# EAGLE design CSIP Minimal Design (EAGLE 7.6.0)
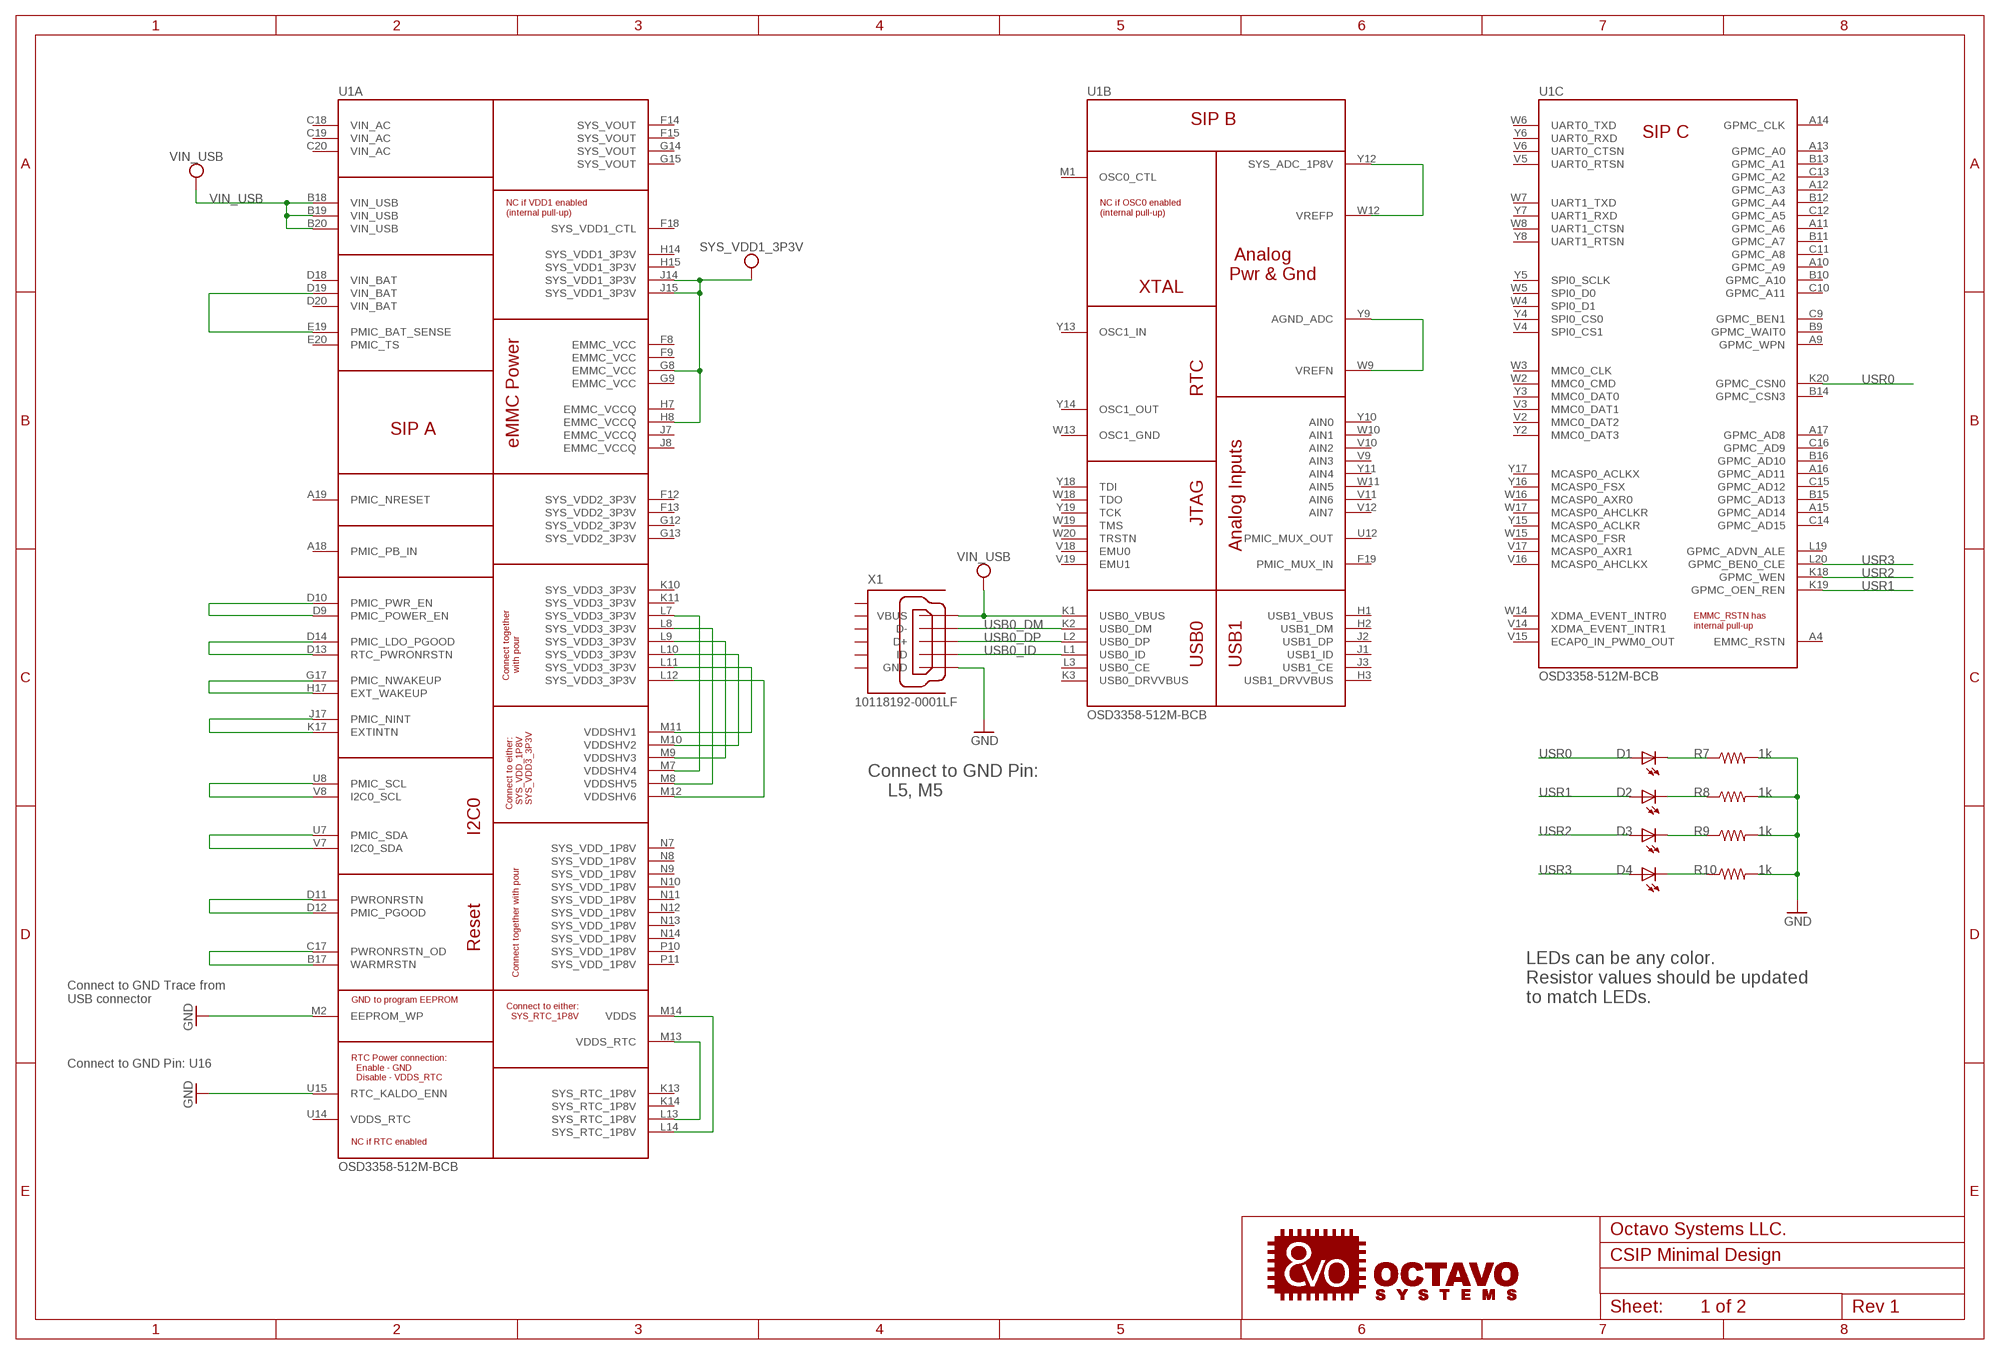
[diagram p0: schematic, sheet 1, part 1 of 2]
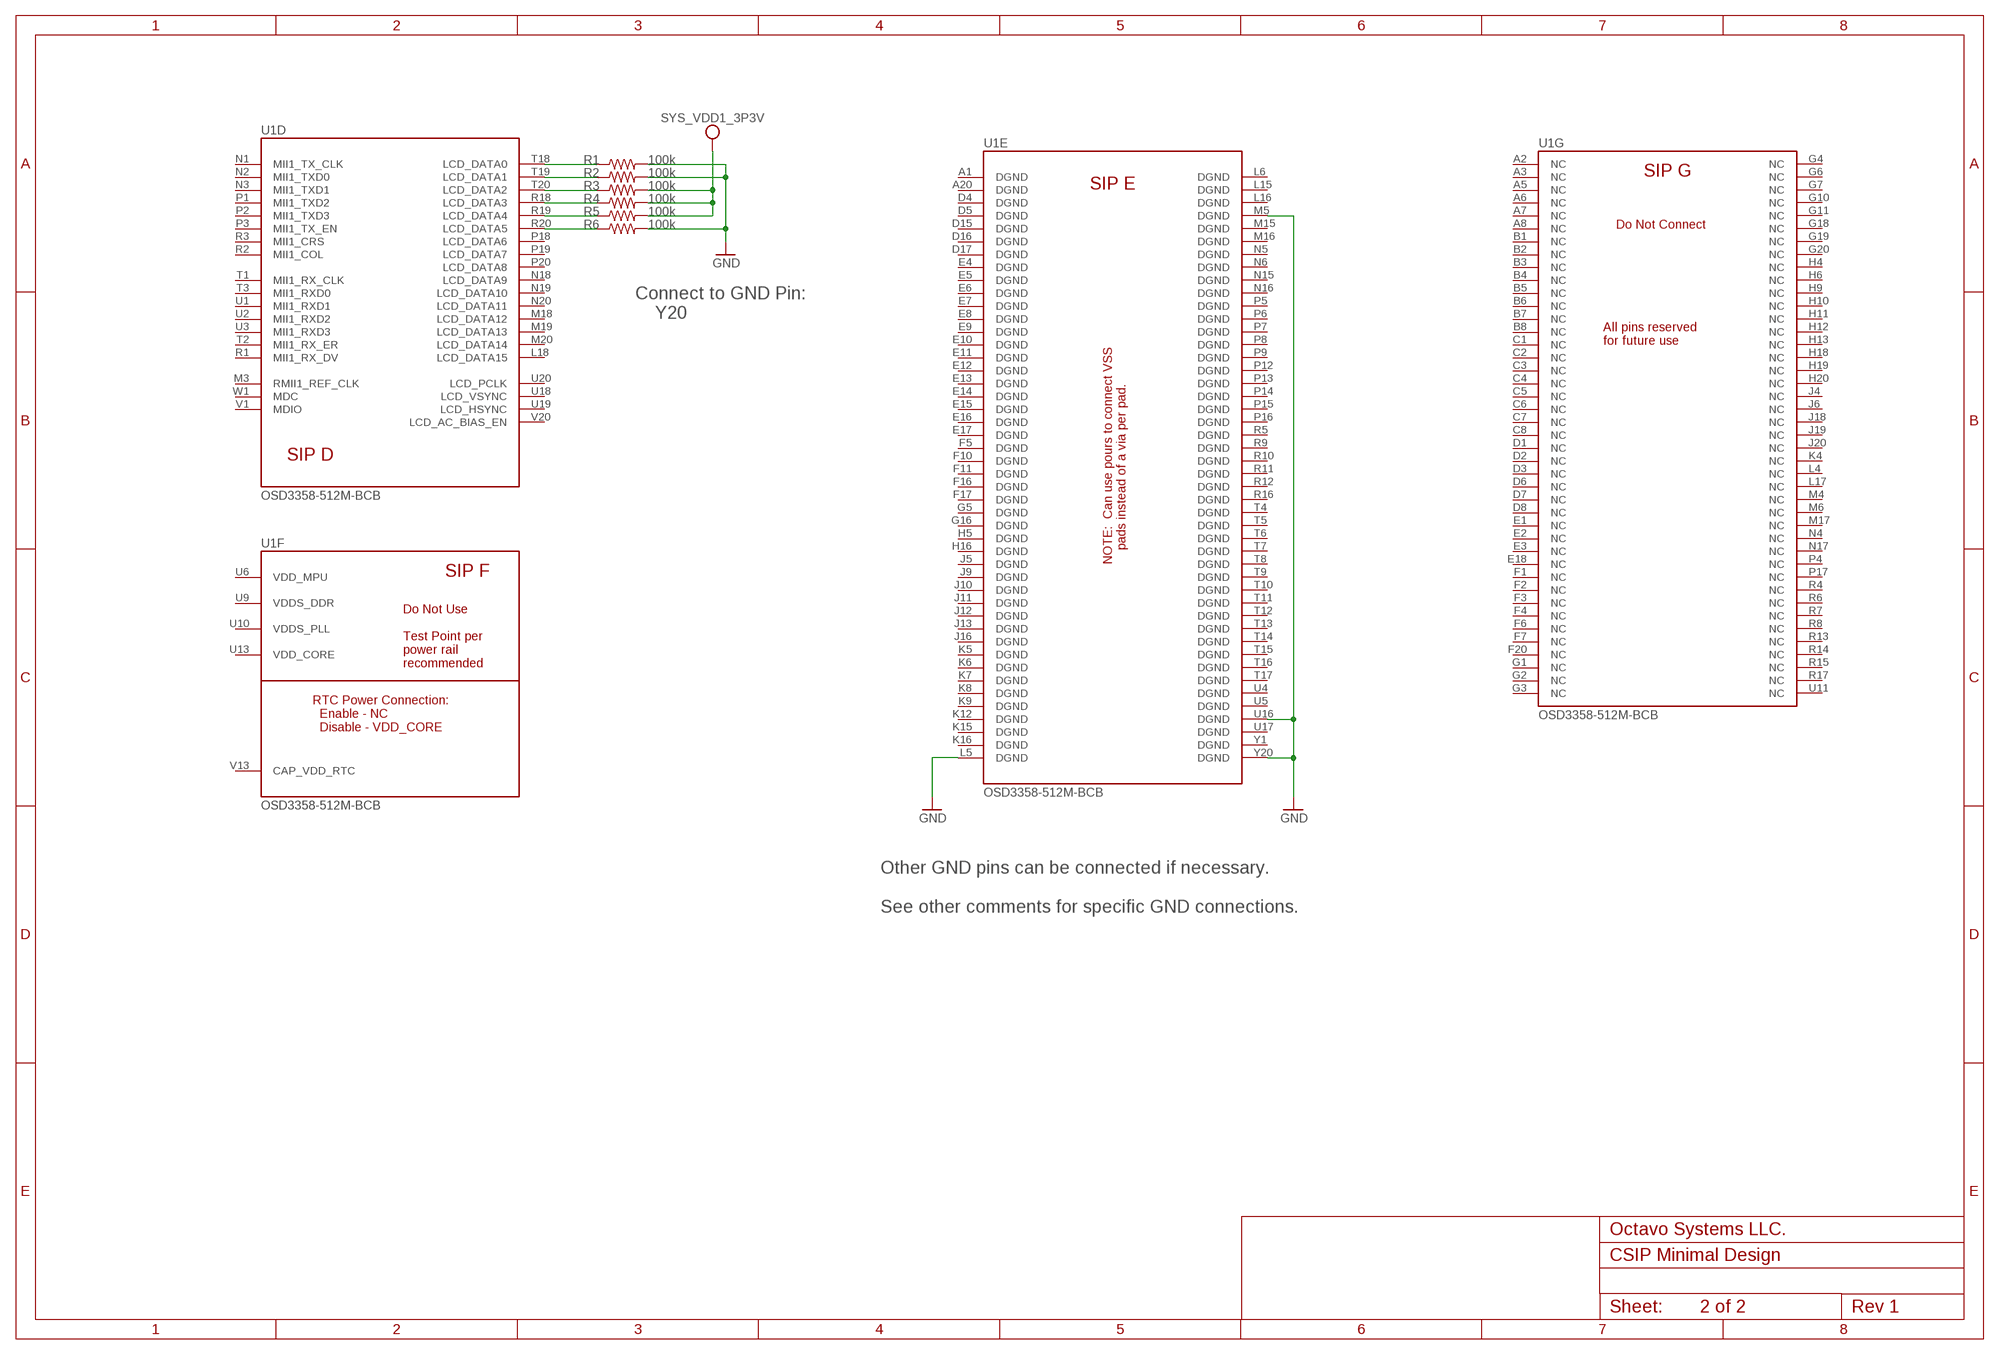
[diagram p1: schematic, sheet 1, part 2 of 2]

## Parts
D1  LTST-C191TBKTLED_EIA-STD  [EIA-STD]
D2  LTST-C191TBKTLED_EIA-STD  [EIA-STD]
D3  LTST-C191TBKTLED_EIA-STD  [EIA-STD]
D4  LTST-C191TBKTLED_EIA-STD  [EIA-STD]
R1  100k  R-US_R0402  [R0402]
R2  100k  R-US_R0402  [R0402]
R3  100k  R-US_R0402  [R0402]
R4  100k  R-US_R0402  [R0402]
R5  100k  R-US_R0402  [R0402]
R6  100k  R-US_R0402  [R0402]
R7  1k  R-US_R0402  [R0402]
R8  1k  R-US_R0402  [R0402]
R9  1k  R-US_R0402  [R0402]
R10  1k  R-US_R0402  [R0402]
U1  OSD3358-512M-BCB  [OSD335X-BGA-400]
X1  10118192-0001LF  [10118192-0001LF(MICRO-USB-B-AMPHENOL-FCI)]

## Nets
GND: R1.2 R2.2 R6.2 R7.2 R8.2 R9.2 R10.2 U1.L5(E:DGND) U1.M2(A:EEPROM_WP) U1.M5(E:DGND) U1.U15(A:RTC_KALDO_ENN) U1.U16(E:DGND) U1.Y20(E:DGND) X1.GND
N$1: U1.G17(A:PMIC_NWAKEUP) U1.H17(A:EXT_WAKEUP)
N$2: U1.D13(A:RTC_PWRONRSTN) U1.D14(A:PMIC_LDO_PGOOD)
N$3: U1.D9(A:PMIC_POWER_EN) U1.D10(A:PMIC_PWR_EN)
N$4: U1.J17(A:PMIC_NINT) U1.K17(A:EXTINTN)
N$5: U1.U8(A:PMIC_SCL) U1.V8(A:I2C0_SCL)
N$6: U1.U7(A:PMIC_SDA) U1.V7(A:I2C0_SDA)
N$7: U1.L13(A:SYS_RTC_1P8V) U1.M13(A:VDDS_RTC)
N$9: U1.D11(A:PWRONRSTN) U1.D12(A:PMIC_PGOOD)
N$10: U1.B17(A:WARMRSTN) U1.C17(A:PWRONRSTN_OD)
N$11: U1.W12(B:VREFP) U1.Y12(B:SYS_ADC_1P8V)
N$13: U1.W9(B:VREFN) U1.Y9(B:AGND_ADC)
N$14: R1.1 U1.T18(D:LCD_DATA0)
N$15: R2.1 U1.T19(D:LCD_DATA1)
N$16: U1.L11(A:SYS_VDD3_3P3V) U1.M11(A:VDDSHV1)
N$17: U1.L10(A:SYS_VDD3_3P3V) U1.M10(A:VDDSHV2)
N$18: R3.1 U1.T20(D:LCD_DATA2)
N$19: R4.1 U1.R18(D:LCD_DATA3)
N$20: R5.1 U1.R19(D:LCD_DATA4)
N$21: R6.1 U1.R20(D:LCD_DATA5)
N$22: U1.L9(A:SYS_VDD3_3P3V) U1.M9(A:VDDSHV3)
N$23: U1.L7(A:SYS_VDD3_3P3V) U1.M7(A:VDDSHV4)
N$24: U1.L8(A:SYS_VDD3_3P3V) U1.M8(A:VDDSHV5)
N$25: D1.2(C) R7.1
N$26: D2.2(C) R8.1
N$27: D3.2(C) R9.1
N$28: D4.2(C) R10.1
SYS_RTC_1P8V: U1.L14(A:SYS_RTC_1P8V) U1.M14(A:VDDS)
SYS_VDD1_3P3V: R3.2 R4.2 R5.2 U1.G8(A:EMMC_VCC) U1.H8(A:EMMC_VCCQ) U1.J14(A:SYS_VDD1_3P3V) U1.J15(A:SYS_VDD1_3P3V)
SYS_VDD3_3P3V: U1.L12(A:SYS_VDD3_3P3V) U1.M12(A:VDDSHV6)
USB0_DM: U1.K2(B:USB0_DM) X1.D-
USB0_DP: U1.L2(B:USB0_DP) X1.D+
USB0_ID: U1.L1(B:USB0_ID) X1.ID
USR0: D1.1(A) U1.K20(C:GPMC_CSN0)
USR1: D2.1(A) U1.K19(C:GPMC_OEN_REN)
USR2: D3.1(A) U1.K18(C:GPMC_WEN)
USR3: D4.1(A) U1.L20(C:GPMC_BEN0_CLE)
VIN_BAT: U1.D19(A:VIN_BAT) U1.E19(A:PMIC_BAT_SENSE)
VIN_USB: U1.B18(A:VIN_USB) U1.B19(A:VIN_USB) U1.B20(A:VIN_USB) U1.K1(B:USB0_VBUS) X1.VBUS
Unconnected: U1.A1(E:DGND) U1.A2(G:NC) U1.A3(G:NC) U1.A4(C:EMMC_RSTN) U1.A5(G:NC) U1.A6(G:NC) U1.A7(G:NC) U1.A8(G:NC) U1.A9(C:GPMC_WPN) U1.A10(C:GPMC_A9) U1.A11(C:GPMC_A6) U1.A12(C:GPMC_A3) U1.A13(C:GPMC_A0) U1.A14(C:GPMC_CLK) U1.A15(C:GPMC_AD14) U1.A16(C:GPMC_AD11) U1.A17(C:GPMC_AD8) U1.A18(A:PMIC_PB_IN) U1.A19(A:PMIC_NRESET) U1.A20(E:DGND) U1.B1(G:NC) U1.B2(G:NC) U1.B3(G:NC) U1.B4(G:NC) U1.B5(G:NC) U1.B6(G:NC) U1.B7(G:NC) U1.B8(G:NC) U1.B9(C:GPMC_WAIT0) U1.B10(C:GPMC_A10) U1.B11(C:GPMC_A7) U1.B12(C:GPMC_A4) U1.B13(C:GPMC_A1) U1.B14(C:GPMC_CSN3) U1.B15(C:GPMC_AD13) U1.B16(C:GPMC_AD10) U1.C1(G:NC) U1.C2(G:NC) U1.C3(G:NC) U1.C4(G:NC) U1.C5(G:NC) U1.C6(G:NC) U1.C7(G:NC) U1.C8(G:NC) U1.C9(C:GPMC_BEN1) U1.C10(C:GPMC_A11) U1.C11(C:GPMC_A8) U1.C12(C:GPMC_A5) U1.C13(C:GPMC_A2) U1.C14(C:GPMC_AD15) U1.C15(C:GPMC_AD12) U1.C16(C:GPMC_AD9) U1.D1(G:NC) U1.D2(G:NC) U1.D3(G:NC) U1.D4(E:DGND) U1.D5(E:DGND) U1.D6(G:NC) U1.D7(G:NC) U1.D8(G:NC) U1.D15(E:DGND) U1.D16(E:DGND) U1.D17(E:DGND) U1.E1(G:NC) U1.E2(G:NC) U1.E3(G:NC) U1.E4(E:DGND) U1.E5(E:DGND) U1.E6(E:DGND) U1.E7(E:DGND) U1.E8(E:DGND) U1.E9(E:DGND) U1.E10(E:DGND) U1.E11(E:DGND) U1.E12(E:DGND) U1.E13(E:DGND) U1.E14(E:DGND) U1.E15(E:DGND) U1.E16(E:DGND) U1.E17(E:DGND) U1.E18(G:NC) U1.E20(A:PMIC_TS) U1.F1(G:NC) U1.F2(G:NC) U1.F3(G:NC) U1.F4(G:NC) U1.F5(E:DGND) U1.F6(G:NC) U1.F7(G:NC) U1.F8(A:EMMC_VCC) U1.F9(A:EMMC_VCC) U1.F10(E:DGND) U1.F11(E:DGND) U1.F16(E:DGND) U1.F17(E:DGND) U1.F18(A:SYS_VDD1_CTL) U1.F19(B:PMIC_MUX_IN) U1.F20(G:NC) U1.G1(G:NC) U1.G2(G:NC) U1.G3(G:NC) U1.G4(G:NC) U1.G5(E:DGND) U1.G6(G:NC) U1.G7(G:NC) U1.G9(A:EMMC_VCC) U1.G10(G:NC) U1.G11(G:NC) U1.G16(E:DGND) U1.G18(G:NC) U1.G19(G:NC) U1.G20(G:NC) U1.H1(B:USB1_VBUS) U1.H2(B:USB1_DM) U1.H3(B:USB1_DRVVBUS) U1.H4(G:NC) U1.H5(E:DGND) U1.H6(G:NC) U1.H7(A:EMMC_VCCQ) U1.H9(G:NC) U1.H10(G:NC) U1.H11(G:NC) U1.H12(G:NC) U1.H13(G:NC) U1.H16(E:DGND) U1.H18(G:NC) U1.H19(G:NC) U1.H20(G:NC) U1.J1(B:USB1_ID) U1.J2(B:USB1_DP) U1.J3(B:USB1_CE) U1.J4(G:NC) U1.J5(E:DGND) U1.J6(G:NC) U1.J7(A:EMMC_VCCQ) U1.J8(A:EMMC_VCCQ) U1.J9(E:DGND) U1.J10(E:DGND) U1.J11(E:DGND) U1.J12(E:DGND) U1.J13(E:DGND) U1.J16(E:DGND) U1.J18(G:NC) U1.J19(G:NC) U1.J20(G:NC) U1.K3(B:USB0_DRVVBUS) U1.K4(G:NC) U1.K5(E:DGND) U1.K6(E:DGND) U1.K7(E:DGND) U1.K8(E:DGND) U1.K9(E:DGND) U1.K12(E:DGND) U1.K15(E:DGND) U1.K16(E:DGND) U1.L3(B:USB0_CE) U1.L4(G:NC) U1.L6(E:DGND) U1.L15(E:DGND) U1.L16(E:DGND) U1.L17(G:NC) U1.L18(D:LCD_DATA15) U1.L19(C:GPMC_ADVN_ALE) U1.M1(B:OSC0_CTL) U1.M3(D:RMII1_REF_CLK) U1.M4(G:NC) U1.M6(G:NC) U1.M15(E:DGND) U1.M16(E:DGND) U1.M17(G:NC) U1.M18(D:LCD_DATA12) U1.M19(D:LCD_DATA13) U1.M20(D:LCD_DATA14) U1.N1(D:MII1_TX_CLK) U1.N2(D:MII1_TXD0) U1.N3(D:MII1_TXD1) U1.N4(G:NC) U1.N5(E:DGND) U1.N6(E:DGND) U1.N15(E:DGND) U1.N16(E:DGND) U1.N17(G:NC) U1.N18(D:LCD_DATA9) U1.N19(D:LCD_DATA10) U1.N20(D:LCD_DATA11) U1.P1(D:MII1_TXD2) U1.P2(D:MII1_TXD3) U1.P3(D:MII1_TX_EN) U1.P4(G:NC) U1.P5(E:DGND) U1.P6(E:DGND) U1.P7(E:DGND) U1.P8(E:DGND) U1.P9(E:DGND) U1.P12(E:DGND) U1.P13(E:DGND) U1.P14(E:DGND) U1.P15(E:DGND) U1.P16(E:DGND) U1.P17(G:NC) U1.P18(D:LCD_DATA6) U1.P19(D:LCD_DATA7) U1.P20(D:LCD_DATA8) U1.R1(D:MII1_RX_DV) U1.R2(D:MII1_COL) U1.R3(D:MII1_CRS) U1.R4(G:NC) U1.R5(E:DGND) U1.R6(G:NC) U1.R7(G:NC) U1.R8(G:NC) U1.R9(E:DGND) U1.R10(E:DGND) U1.R11(E:DGND) U1.R12(E:DGND) U1.R13(G:NC) U1.R14(G:NC) U1.R15(G:NC) U1.R16(E:DGND) U1.R17(G:NC) U1.T1(D:MII1_RX_CLK) U1.T2(D:MII1_RX_ER) U1.T3(D:MII1_RXD0) U1.T4(E:DGND) U1.T5(E:DGND) U1.T6(E:DGND) U1.T7(E:DGND) U1.T8(E:DGND) U1.T9(E:DGND) U1.T10(E:DGND) U1.T11(E:DGND) U1.T12(E:DGND) U1.T13(E:DGND) U1.T14(E:DGND) U1.T15(E:DGND) U1.T16(E:DGND) U1.T17(E:DGND) U1.U1(D:MII1_RXD1) U1.U2(D:MII1_RXD2) U1.U3(D:MII1_RXD3) U1.U4(E:DGND) U1.U5(E:DGND) U1.U6(F:VDD_MPU) U1.U9(F:VDDS_DDR) U1.U10(F:VDDS_PLL) U1.U11(G:NC) U1.U12(B:PMIC_MUX_OUT) U1.U13(F:VDD_CORE) U1.U14(A:VDDS_RTC) U1.U17(E:DGND) U1.U18(D:LCD_VSYNC) U1.U19(D:LCD_HSYNC) U1.U20(D:LCD_PCLK) U1.V1(D:MDIO) U1.V2(C:MMC0_DAT2) U1.V3(C:MMC0_DAT1) U1.V4(C:SPI0_CS1) U1.V5(C:UART0_RTSN) U1.V6(C:UART0_CTSN) U1.V9(B:AIN3) U1.V10(B:AIN2) U1.V11(B:AIN6) U1.V12(B:AIN7) U1.V13(F:CAP_VDD_RTC) U1.V14(C:XDMA_EVENT_INTR1) U1.V15(C:ECAP0_IN_PWM0_OUT) U1.V16(C:MCASP0_AHCLKX) U1.V17(C:MCASP0_AXR1) U1.V18(B:EMU0) U1.V19(B:EMU1) U1.V20(D:LCD_AC_BIAS_EN) U1.W1(D:MDC) U1.W2(C:MMC0_CMD) U1.W3(C:MMC0_CLK) U1.W4(C:SPI0_D1) U1.W5(C:SPI0_D0) U1.W6(C:UART0_TXD) U1.W7(C:UART1_TXD) U1.W8(C:UART1_CTSN) U1.W10(B:AIN1) U1.W11(B:AIN5) U1.W13(B:OSC1_GND) U1.W14(C:XDMA_EVENT_INTR0) U1.W15(C:MCASP0_FSR) U1.W16(C:MCASP0_AXR0) U1.W17(C:MCASP0_AHCLKR) U1.W18(B:TDO) U1.W19(B:TMS) U1.W20(B:TRSTN) U1.Y1(E:DGND) U1.Y2(C:MMC0_DAT3) U1.Y3(C:MMC0_DAT0) U1.Y4(C:SPI0_CS0) U1.Y5(C:SPI0_SCLK) U1.Y6(C:UART0_RXD) U1.Y7(C:UART1_RXD) U1.Y8(C:UART1_RTSN) U1.Y10(B:AIN0) U1.Y11(B:AIN4) U1.Y13(B:OSC1_IN) U1.Y14(B:OSC1_OUT) U1.Y15(C:MCASP0_ACLKR) U1.Y16(C:MCASP0_FSX) U1.Y17(C:MCASP0_ACLKX) U1.Y18(B:TDI) U1.Y19(B:TCK) X1.CGND1(SGND1) X1.CGND2(SGND2) X1.CGND3(SGND3) X1.CGND4(SGND4) X1.CGND5(SGND5) X1.CGND6(SGND6)

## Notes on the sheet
- Connect to GND Pin: 
      Y20
- Connect to GND Pin: 
      L5, M5
- Other GND pins can be connected if necessary.
  
  See other comments for specific GND connections.
- Connect to GND Trace from 
  USB connector
- LEDs can be any color.
  Resistor values should be updated 
  to match LEDs.
- Connect to GND Pin: U16
- 1 of 2 | 2 of 2

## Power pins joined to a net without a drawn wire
SYS_RTC_1P8V: U1.K13(A:SYS_RTC_1P8V) U1.K14(A:SYS_RTC_1P8V)
SYS_VDD1_3P3V: U1.H14(A:SYS_VDD1_3P3V) U1.H15(A:SYS_VDD1_3P3V)
SYS_VDD2_3P3V: U1.F12(A:SYS_VDD2_3P3V) U1.F13(A:SYS_VDD2_3P3V) U1.G12(A:SYS_VDD2_3P3V) U1.G13(A:SYS_VDD2_3P3V)
SYS_VDD3_3P3V: U1.K10(A:SYS_VDD3_3P3V) U1.K11(A:SYS_VDD3_3P3V)
SYS_VDD_1P8V: U1.N7(A:SYS_VDD_1P8V) U1.N8(A:SYS_VDD_1P8V) U1.N9(A:SYS_VDD_1P8V) U1.N10(A:SYS_VDD_1P8V) U1.N11(A:SYS_VDD_1P8V) U1.N12(A:SYS_VDD_1P8V) U1.N13(A:SYS_VDD_1P8V) U1.N14(A:SYS_VDD_1P8V) U1.P10(A:SYS_VDD_1P8V) U1.P11(A:SYS_VDD_1P8V)
SYS_VOUT: U1.F14(A:SYS_VOUT) U1.F15(A:SYS_VOUT) U1.G14(A:SYS_VOUT) U1.G15(A:SYS_VOUT)
VIN_AC: U1.C18(A:VIN_AC) U1.C19(A:VIN_AC) U1.C20(A:VIN_AC)
VIN_BAT: U1.D18(A:VIN_BAT) U1.D20(A:VIN_BAT)

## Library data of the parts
D1-D4 = OSD3358-SM-RED Platform:LTST-C191TBKT: PointLED® Enhanced Thinfilm LED TOP & BOTTOM mount
R1-R10 = OSD3358-SM IOT SoM:R-US_: RESISTOR, American symbol
U1 = Octavo-Systems:OSD3358-512M-BCB: Octavo Systems LLC OSD335x Family SiP: 27mm x 27mm, 1.27mm pitch 400 pin BGA contains AM3358, 512MB DDR3, TPS65217, TL5209, 4KB EEPROM, 4GB eMMC, 24MHz oscillator, and passives. Commerical Temperature (case): 0C to 85C.
X1 = OSD3358-SM-RED Platform:10118192-0001LF: Amphenol FCI Micro USB Type B Complete Surface Mount (SMT) no guide holes

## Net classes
1 ground: width 0.152 mm, drill 0.254 mm, clearance 0.152 mm
3 power: width 0.152 mm, drill 0.254 mm, clearance 0.152 mm

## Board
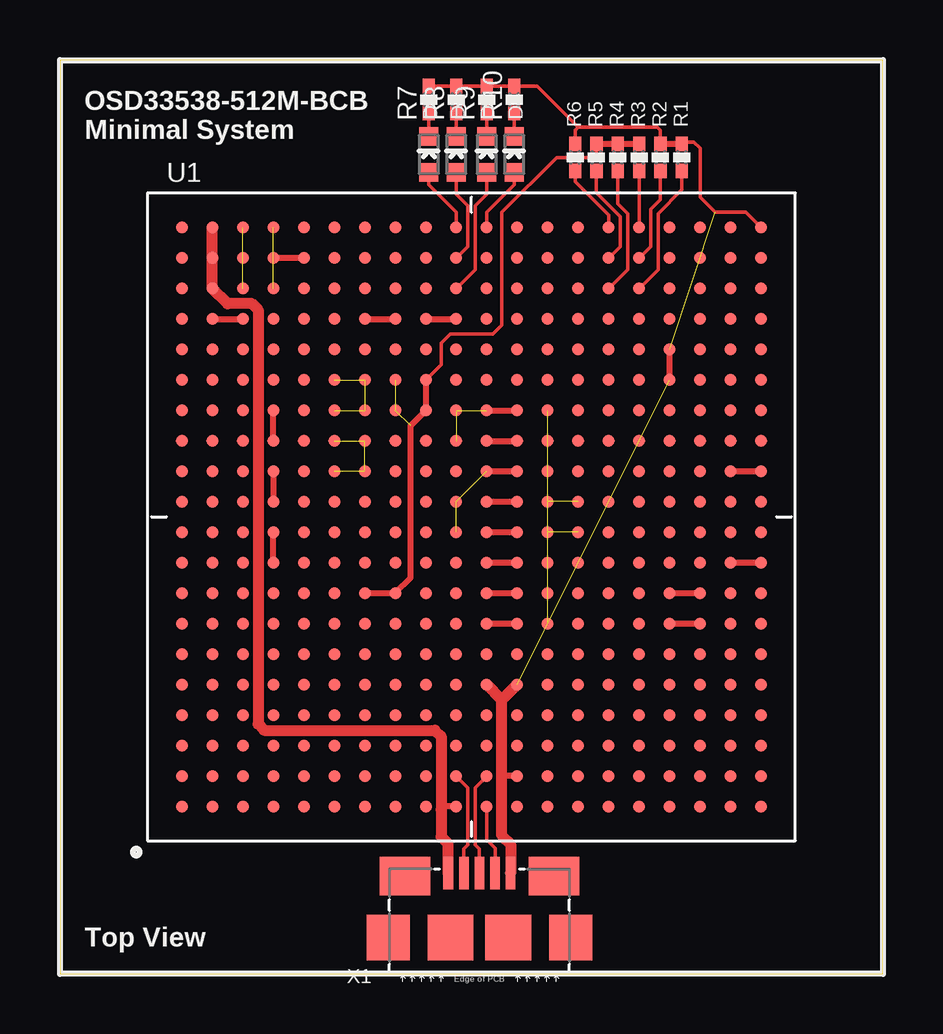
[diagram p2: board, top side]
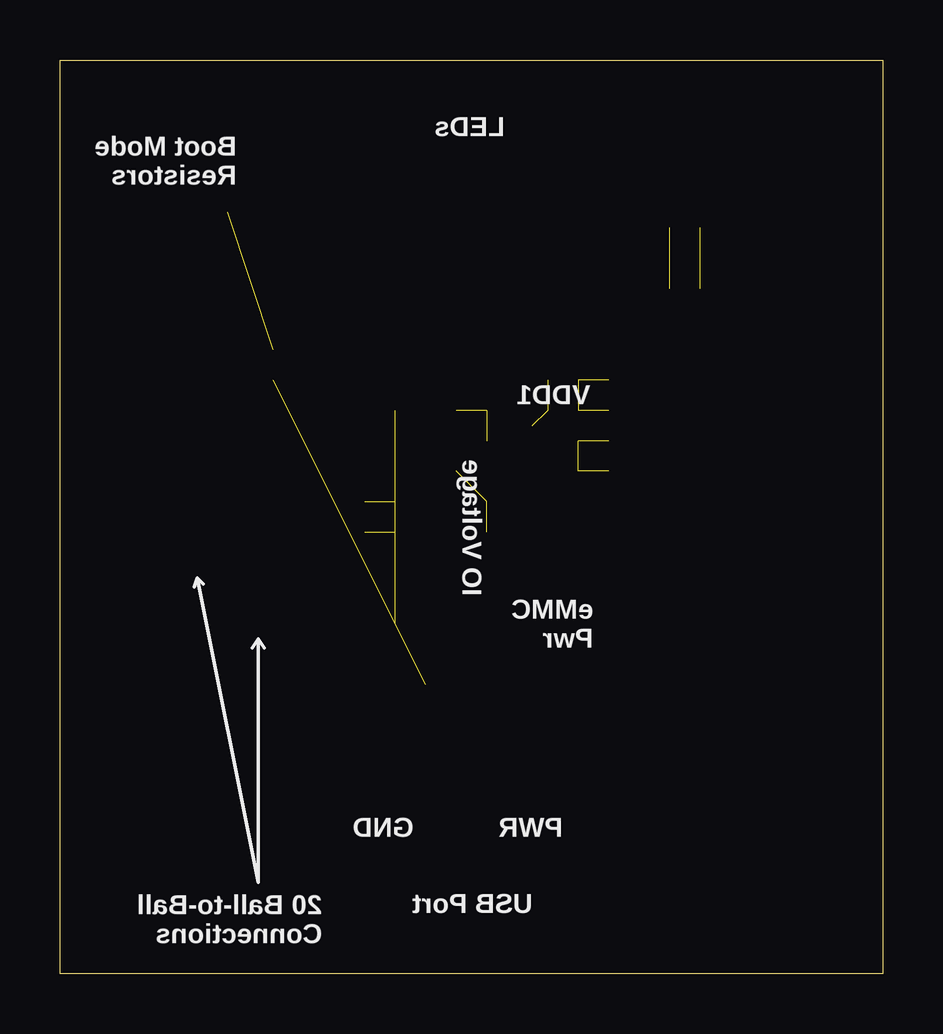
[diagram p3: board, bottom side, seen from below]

Size 34.29 x 38.1 mm. Coordinates in mm from the lower left corner, seen from the top.
Outline: 0,0 34.29,0 34.29,38.1 0,38.1 0,0
Copper layers (1*16): Top 0.035mm / dielectric 1.5mm / Bottom 0.035mm
Design rules "default *": minimum track width 6mil, minimum drill 10mil, track to track 6mil, track to pad 6mil, pad to pad 6mil, via to via 6mil, smd to smd 6mil, copper to edge 10mil, drill to drill 8mil, minimum pad ring 10mil, minimum via ring 5mil, stop-mask expansion 3mil, vias tented up to drill 40mil, thermal gap 10mil

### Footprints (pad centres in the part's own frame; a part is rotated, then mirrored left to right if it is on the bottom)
EIA-STD = smd 0.787 x 0.787: 1 -0.749,0; 2 0.749,0
R0402 = smd 0.61 x 0.508: 1 -0.559,0; 2 0.559,0
OSD335X-BGA-400 = smd 0.5 x 0.5: A1 -12.065,-12.065; A2 -12.065,-10.795; A3 -12.065,-9.525; A4 -12.065,-8.255; A5 -12.065,-6.985; A6 -12.065,-5.715; A7 -12.065,-4.445; A8 -12.065,-3.175; A9 -12.065,-1.905; A10 -12.065,-0.635; A11 -12.065,0.635; A12 -12.065,1.905; A13 -12.065,3.175; A14 -12.065,4.445; A15 -12.065,5.715; A16 -12.065,6.985; A17 -12.065,8.255; A18 -12.065,9.525; A19 -12.065,10.795; A20 -12.065,12.065; B1 -10.795,-12.065; B2 -10.795,-10.795; B3 -10.795,-9.525; B4 -10.795,-8.255; B5 -10.795,-6.985; B6 -10.795,-5.715; B7 -10.795,-4.445; B8 -10.795,-3.175; B9 -10.795,-1.905; B10 -10.795,-0.635; B11 -10.795,0.635; B12 -10.795,1.905; B13 -10.795,3.175; B14 -10.795,4.445; B15 -10.795,5.715; B16 -10.795,6.985; B17 -10.795,8.255; B18 -10.795,9.525; B19 -10.795,10.795; B20 -10.795,12.065; C1 -9.525,-12.065; C2 -9.525,-10.795; C3 -9.525,-9.525; C4 -9.525,-8.255; C5 -9.525,-6.985; C6 -9.525,-5.715; C7 -9.525,-4.445; C8 -9.525,-3.175; C9 -9.525,-1.905; C10 -9.525,-0.635; C11 -9.525,0.635; C12 -9.525,1.905; C13 -9.525,3.175; C14 -9.525,4.445; C15 -9.525,5.715; C16 -9.525,6.985; C17 -9.525,8.255; C18 -9.525,9.525; C19 -9.525,10.795; C20 -9.525,12.065; D1 -8.255,-12.065; D2 -8.255,-10.795; D3 -8.255,-9.525; D4 -8.255,-8.255; D5 -8.255,-6.985; D6 -8.255,-5.715; D7 -8.255,-4.445; D8 -8.255,-3.175; D9 -8.255,-1.905; D10 -8.255,-0.635; D11 -8.255,0.635; D12 -8.255,1.905; D13 -8.255,3.175; D14 -8.255,4.445; D15 -8.255,5.715; D16 -8.255,6.985; D17 -8.255,8.255; D18 -8.255,9.525; D19 -8.255,10.795; D20 -8.255,12.065; E1 -6.985,-12.065; E2 -6.985,-10.795; E3 -6.985,-9.525; E4 -6.985,-8.255; E5 -6.985,-6.985; E6 -6.985,-5.715; E7 -6.985,-4.445; E8 -6.985,-3.175; E9 -6.985,-1.905; E10 -6.985,-0.635; E11 -6.985,0.635; E12 -6.985,1.905; E13 -6.985,3.175; E14 -6.985,4.445; E15 -6.985,5.715; E16 -6.985,6.985; E17 -6.985,8.255; E18 -6.985,9.525; E19 -6.985,10.795; E20 -6.985,12.065; F1 -5.715,-12.065; F2 -5.715,-10.795; F3 -5.715,-9.525; F4 -5.715,-8.255; F5 -5.715,-6.985; F6 -5.715,-5.715; F7 -5.715,-4.445; F8 -5.715,-3.175; F9 -5.715,-1.905; F10 -5.715,-0.635; F11 -5.715,0.635; F12 -5.715,1.905; F13 -5.715,3.175; F14 -5.715,4.445; F15 -5.715,5.715; F16 -5.715,6.985; F17 -5.715,8.255; F18 -5.715,9.525; F19 -5.715,10.795; F20 -5.715,12.065; G1 -4.445,-12.065; G2 -4.445,-10.795; G3 -4.445,-9.525; G4 -4.445,-8.255; G5 -4.445,-6.985; G6 -4.445,-5.715; G7 -4.445,-4.445; G8 -4.445,-3.175; G9 -4.445,-1.905; G10 -4.445,-0.635; G11 -4.445,0.635; G12 -4.445,1.905; G13 -4.445,3.175; G14 -4.445,4.445; G15 -4.445,5.715; G16 -4.445,6.985; G17 -4.445,8.255; G18 -4.445,9.525; G19 -4.445,10.795; G20 -4.445,12.065; H1 -3.175,-12.065; H2 -3.175,-10.795; H3 -3.175,-9.525; H4 -3.175,-8.255; H5 -3.175,-6.985; H6 -3.175,-5.715; H7 -3.175,-4.445; H8 -3.175,-3.175; H9 -3.175,-1.905; H10 -3.175,-0.635; H11 -3.175,0.635; H12 -3.175,1.905; H13 -3.175,3.175; H14 -3.175,4.445; H15 -3.175,5.715; H16 -3.175,6.985; H17 -3.175,8.255; H18 -3.175,9.525; H19 -3.175,10.795; H20 -3.175,12.065; J1 -1.905,-12.065; J2 -1.905,-10.795; J3 -1.905,-9.525; J4 -1.905,-8.255; J5 -1.905,-6.985; J6 -1.905,-5.715; J7 -1.905,-4.445; J8 -1.905,-3.175; J9 -1.905,-1.905; J10 -1.905,-0.635; J11 -1.905,0.635; J12 -1.905,1.905; J13 -1.905,3.175; J14 -1.905,4.445; J15 -1.905,5.715; J16 -1.905,6.985; J17 -1.905,8.255; J18 -1.905,9.525; J19 -1.905,10.795; J20 -1.905,12.065; K1 -0.635,-12.065; K2 -0.635,-10.795; K3 -0.635,-9.525; K4 -0.635,-8.255; K5 -0.635,-6.985; K6 -0.635,-5.715; K7 -0.635,-4.445; K8 -0.635,-3.175; K9 -0.635,-1.905; K10 -0.635,-0.635; K11 -0.635,0.635; K12 -0.635,1.905; K13 -0.635,3.175; K14 -0.635,4.445; K15 -0.635,5.715; K16 -0.635,6.985; K17 -0.635,8.255; K18 -0.635,9.525; K19 -0.635,10.795; K20 -0.635,12.065; L1 0.635,-12.065; L2 0.635,-10.795; L3 0.635,-9.525; L4 0.635,-8.255; L5 0.635,-6.985; L6 0.635,-5.715; L7 0.635,-4.445; L8 0.635,-3.175; L9 0.635,-1.905; L10 0.635,-0.635; L11 0.635,0.635; L12 0.635,1.905; L13 0.635,3.175; L14 0.635,4.445; L15 0.635,5.715; L16 0.635,6.985; L17 0.635,8.255; L18 0.635,9.525; L19 0.635,10.795; L20 0.635,12.065; M1 1.905,-12.065; M2 1.905,-10.795; M3 1.905,-9.525; M4 1.905,-8.255; M5 1.905,-6.985; M6 1.905,-5.715; M7 1.905,-4.445; M8 1.905,-3.175; M9 1.905,-1.905; M10 1.905,-0.635; M11 1.905,0.635; M12 1.905,1.905; M13 1.905,3.175; M14 1.905,4.445; M15 1.905,5.715; M16 1.905,6.985; M17 1.905,8.255; M18 1.905,9.525; M19 1.905,10.795; M20 1.905,12.065; N1 3.175,-12.065; N2 3.175,-10.795; N3 3.175,-9.525; N4 3.175,-8.255; N5 3.175,-6.985; N6 3.175,-5.715; N7 3.175,-4.445; N8 3.175,-3.175; N9 3.175,-1.905; N10 3.175,-0.635; N11 3.175,0.635; N12 3.175,1.905; N13 3.175,3.175; N14 3.175,4.445; N15 3.175,5.715; N16 3.175,6.985; N17 3.175,8.255; N18 3.175,9.525; N19 3.175,10.795; N20 3.175,12.065; P1 4.445,-12.065; P2 4.445,-10.795; P3 4.445,-9.525; P4 4.445,-8.255; P5 4.445,-6.985; P6 4.445,-5.715; P7 4.445,-4.445; P8 4.445,-3.175; P9 4.445,-1.905; P10 4.445,-0.635; P11 4.445,0.635; P12 4.445,1.905; P13 4.445,3.175; P14 4.445,4.445; P15 4.445,5.715; P16 4.445,6.985; P17 4.445,8.255; P18 4.445,9.525; P19 4.445,10.795; P20 4.445,12.065; R1 5.715,-12.065; R2 5.715,-10.795; R3 5.715,-9.525; R4 5.715,-8.255; R5 5.715,-6.985; R6 5.715,-5.715; R7 5.715,-4.445; R8 5.715,-3.175; R9 5.715,-1.905; R10 5.715,-0.635; R11 5.715,0.635; R12 5.715,1.905; R13 5.715,3.175; R14 5.715,4.445; R15 5.715,5.715; R16 5.715,6.985; R17 5.715,8.255; R18 5.715,9.525; R19 5.715,10.795; R20 5.715,12.065; T1 6.985,-12.065; T2 6.985,-10.795; T3 6.985,-9.525; T4 6.985,-8.255; T5 6.985,-6.985; T6 6.985,-5.715; T7 6.985,-4.445; T8 6.985,-3.175; T9 6.985,-1.905; T10 6.985,-0.635; T11 6.985,0.635; T12 6.985,1.905; T13 6.985,3.175; T14 6.985,4.445; T15 6.985,5.715; T16 6.985,6.985; T17 6.985,8.255; T18 6.985,9.525; T19 6.985,10.795; T20 6.985,12.065; U1 8.255,-12.065; U2 8.255,-10.795; U3 8.255,-9.525; U4 8.255,-8.255; U5 8.255,-6.985; U6 8.255,-5.715; U7 8.255,-4.445; U8 8.255,-3.175; U9 8.255,-1.905; U10 8.255,-0.635; U11 8.255,0.635; U12 8.255,1.905; U13 8.255,3.175; U14 8.255,4.445; U15 8.255,5.715; U16 8.255,6.985; U17 8.255,8.255; U18 8.255,9.525; U19 8.255,10.795; U20 8.255,12.065; V1 9.525,-12.065; V2 9.525,-10.795; V3 9.525,-9.525; V4 9.525,-8.255; V5 9.525,-6.985; V6 9.525,-5.715; V7 9.525,-4.445; V8 9.525,-3.175; V9 9.525,-1.905; V10 9.525,-0.635; V11 9.525,0.635; V12 9.525,1.905; V13 9.525,3.175; V14 9.525,4.445; V15 9.525,5.715; V16 9.525,6.985; V17 9.525,8.255; V18 9.525,9.525; V19 9.525,10.795; V20 9.525,12.065; W1 10.795,-12.065; W2 10.795,-10.795; W3 10.795,-9.525; W4 10.795,-8.255; W5 10.795,-6.985; W6 10.795,-5.715; W7 10.795,-4.445; W8 10.795,-3.175; W9 10.795,-1.905; W10 10.795,-0.635; W11 10.795,0.635; W12 10.795,1.905; W13 10.795,3.175; W14 10.795,4.445; W15 10.795,5.715; W16 10.795,6.985; W17 10.795,8.255; W18 10.795,9.525; W19 10.795,10.795; W20 10.795,12.065; Y1 12.065,-12.065; Y2 12.065,-10.795; Y3 12.065,-9.525; Y4 12.065,-8.255; Y5 12.065,-6.985; Y6 12.065,-5.715; Y7 12.065,-4.445; Y8 12.065,-3.175; Y9 12.065,-1.905; Y10 12.065,-0.635; Y11 12.065,0.635; Y12 12.065,1.905; Y13 12.065,3.175; Y14 12.065,4.445; Y15 12.065,5.715; Y16 12.065,6.985; Y17 12.065,8.255; Y18 12.065,9.525; Y19 12.065,10.795; Y20 12.065,12.065
10118192-0001LF(MICRO-USB-B-AMPHENOL-FCI) = smd 1.8 x 1.9: CGND1 -3.8,0; CGND4 3.8,0 | smd 1.9 x 1.9: CGND2 -1.2,0; CGND3 1.2,0 | smd 2.1 x 1.6: CGND5 3.1,2.55; CGND6 -3.1,2.55 | smd 0.4 x 1.35: D+ 0,2.675; D- -0.65,2.675; GND 1.3,2.675; ID 0.65,2.675; VBUS -1.3,2.675

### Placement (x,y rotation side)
D1  15.37,34.16 90 top
D2  16.51,34.16 90 top
D3  17.78,34.16 90 top
D4  18.92,34.16 90 top
R1  25.91,34.04 90 top
R2  25.02,34.04 90 top
R3  24.13,34.04 90 top
R4  23.24,34.04 90 top
R5  22.35,34.04 90 top
R6  21.46,34.04 90 top
R7  15.37,36.45 90 top
R8  16.51,36.45 90 top
R9  17.78,36.45 90 top
R10  18.92,36.45 90 top
U1  17.14,19.05 0 top
X1  17.48,1.52 0 top

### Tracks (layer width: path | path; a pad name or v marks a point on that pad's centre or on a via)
GND  (2 unrouted)
  Top 0.152: R1.2 25.98,34.67 26.42,34.67 26.67,34.42 26.67,32.38 27.3,31.75 28.57,31.75 U1.Y20 | R6.2 21.46,35.18 21.59,35.31 | 21.59,35.31 24.89,35.31 25.02,35.18 R2.2 | R7.2 R8.2 R9.2 R10.2 19.89,37.01 21.59,35.31
  Top 0.254: R1.2 R2.2 | U1.U15 U1.U16 | U1.M2 18.41,8.26
  Top 0.457: 18.41,11.43 18.41,8.26 18.41,5.76 18.77,5.4 X1.GND | 18.41,11.43 U1.L5 | U1.M5 18.41,11.43
N$1
  Top 0.254: U1.G17 U1.H17
N$2
  Top 0.254: U1.D13 U1.D14
N$3
  Top 0.254: U1.D9 U1.D10
N$4
  Top 0.254: U1.J17 U1.K17
N$5
  Top 0.254: U1.U8 U1.V8
N$6
  Top 0.254: U1.U7 U1.V7
N$7
  Top 0.254: U1.L13 U1.M13
N$9
  Top 0.254: U1.D12 U1.D11
N$10
  Top 0.254: U1.B17 U1.C17
N$11
  Top 0.254: U1.W12 U1.Y12
N$13
  Top 0.254: U1.W9 U1.Y9
N$14
  Top 0.152: U1.T18 24.92,29.36 24.92,31.7 25.91,32.69 R1.1
N$15
  Top 0.152: U1.T19 24.61,30.33 24.61,31.88 25.02,32.28 R2.1
N$16
  Top 0.254: U1.L11 U1.M11
N$17
  Top 0.254: U1.L10 U1.M10
N$18
  Top 0.152: U1.T20 R3.1
N$19
  Top 0.152: U1.R18 23.65,29.36 23.65,31.7 23.24,32.11 R4.1
N$20
  Top 0.152: U1.R19 23.34,30.33 23.34,31.57 22.35,32.56 R5.1
N$21
  Top 0.152: U1.R20 22.86,31.62 21.46,33.02 R6.1
N$22
  Top 0.254: U1.L9 U1.M9
N$23
  Top 0.254: U1.L7 U1.M7
N$24
  Top 0.254: U1.L8 U1.M8
N$25
  Top 0.152: R7.1 D1.2
N$26
  Top 0.152: R8.1 D2.2
N$27
  Top 0.152: R9.1 D3.2
N$28
  Top 0.152: R10.1 D4.2
SYS_RTC_1P8V  (2 unrouted)
  Top 0.254: U1.L14 U1.M14
SYS_VDD1_3P3V  (2 unrouted)
  Top 0.152: R5.2 22.35,34.16 22.23,34.04 20.7,34.04 18.41,31.75 18.41,27.05 18.03,26.67 16.26,26.67 15.88,26.29 15.88,25.4 U1.J15
  Top 0.254: U1.G8 U1.H8 14.61,16.51 14.61,22.86 U1.J14 U1.J15 | R3.2 R4.2 R5.2
SYS_VDD2_3P3V  (3 unrouted)
SYS_VDD3_3P3V  (2 unrouted)
  Top 0.254: U1.L12 U1.M12
SYS_VDD_1P8V  (9 unrouted)
SYS_VOUT  (3 unrouted)
USB0_DM
  Top 0.152: U1.K2 16.51,8.23 16.99,7.75 16.99,5.38 16.82,5.22 X1.D-
USB0_DP
  Top 0.152: U1.L2 17.78,8.23 17.3,7.75 17.3,5.38 17.48,5.21 X1.D+
USB0_ID
  Top 0.152: U1.L1 17.78,5.59 18.12,5.24 X1.ID
USR0
  Top 0.152: U1.K20 16.51,31.75 15.37,32.89 D1.1
USR1
  Top 0.152: D2.1 16.51,32.51 16.99,32.03 16.99,30.33 U1.K19
USR2
  Top 0.152: U1.K18 17.3,29.36 17.3,32.03 17.78,32.51 D3.1
USR3
  Top 0.152: U1.L20 17.78,31.75 18.92,32.89 D4.1
VIN_AC  (2 unrouted)
VIN_BAT  (2 unrouted)
  Top 0.254: U1.E19 U1.D19
VIN_USB
  Top 0.254: X1.VBUS | U1.K1 16,6.99 15.88,6.86
  Top 0.457: X1.VBUS 16.18,5.42 15.88,5.71 15.88,6.86 15.88,9.91 15.62,10.16 8.51,10.16 8.26,10.41 8.26,27.69 8,27.94 6.99,27.94 U1.B18 U1.B19 U1.B20

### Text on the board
tPlace: OSD33538-512M-BCB / Minimal System | Top View
bPlace: LEDs | Boot Mode / Resistors | VDD1 | IO Voltage | eMMC / Pwr | PWR | GND | USB Port | 20 Ball-to-Ball / Connections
